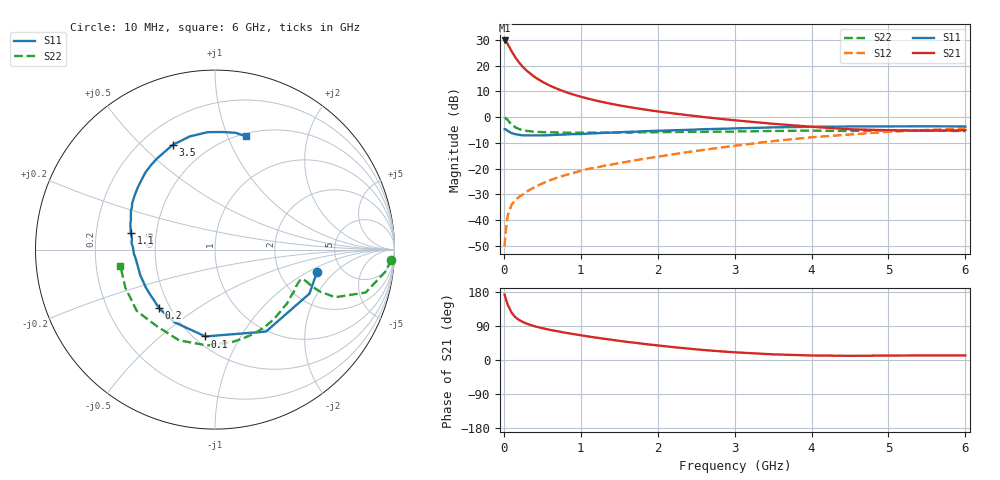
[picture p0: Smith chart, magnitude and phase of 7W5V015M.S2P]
! Infineon Technologies  Discrete & RF Semiconductors
! BFS17W
! Si NPN RF Bipolar Junction Transistor in SOT323
! VCE = 5 V  IC = 15 mA
! Common Emitter S-Parameters:  August  1999
# GHz  S  MA  R  50
!  f  S11  S21  S12  S22
! GHz  MAG  ANG  MAG  ANG  MAG  ANG  MAG  ANG
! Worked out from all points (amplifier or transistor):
!   36 points, 10 MHz to 6 GHz, reference 50 ohm
!   highest |S21| = 29.8 dB at 10 MHz (marker M1)
!   |S21| within 3 dB of that: start of sweep to 79.24 MHz
!   unconditionally stable (mu >= 1): 343.3 MHz to 2.212 GHz; 5.213 GHz to end of sweep
!   at 250 MHz: K = 0.91, MSG = 24.7 dB, |S12| = -30.0 dB
!   at 1.4 GHz: K = 1.18, MAG = 9.3 dB, |S12| = -18.5 dB
!   at 6 GHz: K = 1.05, MAG = -1.7 dB, |S12| = -4.4 dB
!   S11 on the Smith chart (normalised r, x): 10 MHz: 3.26, -1.25; 100 MHz: 0.57, -0.72; 200 MHz: 0.44, -0.36; 1.1 GHz: 0.36, +0.09; 3.5 GHz: 0.32, +0.62; 6 GHz: 0.53, +1.16
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0.01  0.5816 -12.6  30.73 172.6  0.0031 83.0  0.9839 -3.3
0.02  0.5806 -25.0  29.95 164.9  0.0053 83.3  0.957 -7.4
0.05  0.5379 -58.1  26.14 145.8  0.0121 70.0  0.8728 -15.9
0.1  0.4867 -96.4  19.09 125.2  0.0197 60.1  0.7208 -21.6
0.15  0.4637 -119.6  14.37 112.9  0.0247 55.8  0.631 -21.8
0.2  0.4509 -133.6  11.37 105.4  0.0282 59.0  0.583 -20.9
0.25  0.4401 -143.7  9.317 99.9  0.0315 58.7  0.5531 -19.8
0.3  0.4396 -150.7  7.877 95.7  0.0359 61.4  0.5377 -19.2
0.4  0.4401 -161.1  6.009 89.0  0.0436 63.1  0.5172 -18.6
0.5  0.4399 -167.9  4.848 84.0  0.0512 65.0  0.5092 -18.8
0.6  0.4442 -173.0  4.051 79.6  0.0593 66.6  0.5039 -19.7
0.7  0.4526 -177.2  3.5 75.7  0.0669 68.0  0.5004 -21.0
0.9  0.4666 175.3  2.744 68.6  0.082 69.4  0.4965 -24.2
1.1  0.4779 168.8  2.266 62.0  0.0984 69.4  0.4976 -28.3
1.3  0.4931 163.0  1.933 56.1  0.1125 70.2  0.4974 -32.8
1.6  0.5154 155.3  1.586 47.9  0.1352 71.0  0.4995 -40.0
2.2  0.5525 141.1  1.178 34.0  0.1886 71.8  0.511 -56.1
2.8  0.5902 127.2  0.928 23.1  0.2527 69.8  0.5193 -73.5
3.5  0.6291 112.1  0.74 14.9  0.3409 64.6  0.5361 -94.5
4.5  0.6556 93.6  0.579 11.0  0.4578 52.1  0.5358 -127.2
5.5  0.6607 80.1  0.543 12.1  0.56 39.1  0.5428 -156.9
6  0.6544 74.8  0.553 12.1  0.6005 32.7  0.5348 -170.0
